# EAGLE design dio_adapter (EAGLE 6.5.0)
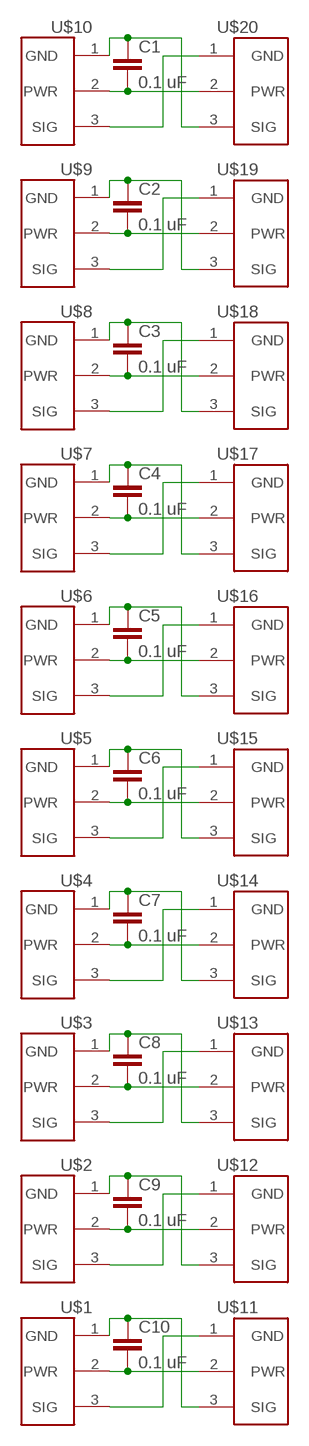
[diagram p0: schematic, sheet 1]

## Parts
C1  0.1 uF  CAP0603  [0603]
C2  0.1 uF  CAP0603  [0603]
C3  0.1 uF  CAP0603  [0603]
C4  0.1 uF  CAP0603  [0603]
C5  0.1 uF  CAP0603  [0603]
C6  0.1 uF  CAP0603  [0603]
C7  0.1 uF  CAP0603  [0603]
C8  0.1 uF  CAP0603  [0603]
C9  0.1 uF  CAP0603  [0603]
C10  0.1 uF  CAP0603  [0603]
U$1  22-23-2031GENERIC  [PWM_1X3]
U$2  22-23-2031GENERIC  [PWM_1X3]
U$3  22-23-2031GENERIC  [PWM_1X3]
U$4  22-23-2031GENERIC  [PWM_1X3]
U$5  22-23-2031GENERIC  [PWM_1X3]
U$6  22-23-2031GENERIC  [PWM_1X3]
U$7  22-23-2031GENERIC  [PWM_1X3]
U$8  22-23-2031GENERIC  [PWM_1X3]
U$9  22-23-2031GENERIC  [PWM_1X3]
U$10  22-23-2031GENERIC  [PWM_1X3]
U$11  22-23-2031  [22-23-2031]
U$12  22-23-2031  [22-23-2031]
U$13  22-23-2031  [22-23-2031]
U$14  22-23-2031  [22-23-2031]
U$15  22-23-2031  [22-23-2031]
U$16  22-23-2031  [22-23-2031]
U$17  22-23-2031  [22-23-2031]
U$18  22-23-2031  [22-23-2031]
U$19  22-23-2031  [22-23-2031]
U$20  22-23-2031  [22-23-2031]

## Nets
N$1: C1.1 U$10.1(GND) U$20.3(SIG)
N$2: C1.2 U$10.2(PWR) U$20.2(PWR)
N$3: U$10.3(SIG) U$20.1(GND)
N$4: C10.1 U$1.1(GND) U$11.3(SIG)
N$5: C2.2 U$9.2(PWR) U$19.2(PWR)
N$6: U$9.3(SIG) U$19.1(GND)
N$7: C9.1 U$2.1(GND) U$12.3(SIG)
N$8: C3.2 U$8.2(PWR) U$18.2(PWR)
N$9: U$8.3(SIG) U$18.1(GND)
N$10: C8.1 U$3.1(GND) U$13.3(SIG)
N$11: C4.2 U$7.2(PWR) U$17.2(PWR)
N$12: U$7.3(SIG) U$17.1(GND)
N$13: C7.1 U$4.1(GND) U$14.3(SIG)
N$14: C5.2 U$6.2(PWR) U$16.2(PWR)
N$15: U$6.3(SIG) U$16.1(GND)
N$16: C6.1 U$5.1(GND) U$15.3(SIG)
N$17: C6.2 U$5.2(PWR) U$15.2(PWR)
N$18: U$5.3(SIG) U$15.1(GND)
N$19: C5.1 U$6.1(GND) U$16.3(SIG)
N$20: C7.2 U$4.2(PWR) U$14.2(PWR)
N$21: U$4.3(SIG) U$14.1(GND)
N$22: C4.1 U$7.1(GND) U$17.3(SIG)
N$23: C8.2 U$3.2(PWR) U$13.2(PWR)
N$24: U$3.3(SIG) U$13.1(GND)
N$25: C3.1 U$8.1(GND) U$18.3(SIG)
N$26: C9.2 U$2.2(PWR) U$12.2(PWR)
N$27: U$2.3(SIG) U$12.1(GND)
N$28: C2.1 U$9.1(GND) U$19.3(SIG)
N$29: C10.2 U$1.2(PWR) U$11.2(PWR)
N$30: U$1.3(SIG) U$11.1(GND)

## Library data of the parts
C1-C10 = custom:CAP: Capacitor
U$1-U$20 = custom:22-23-2031: Molex 3-pin male connector 22-23-2031.

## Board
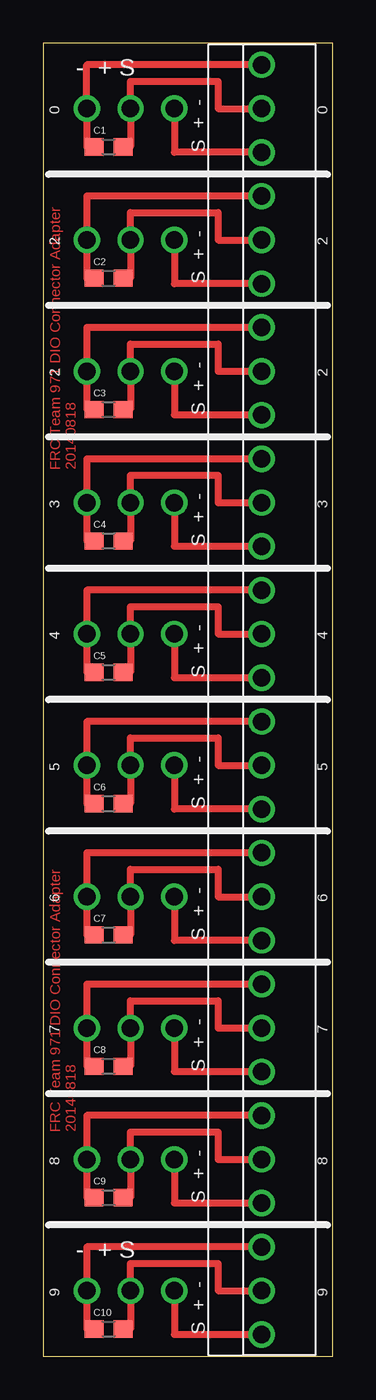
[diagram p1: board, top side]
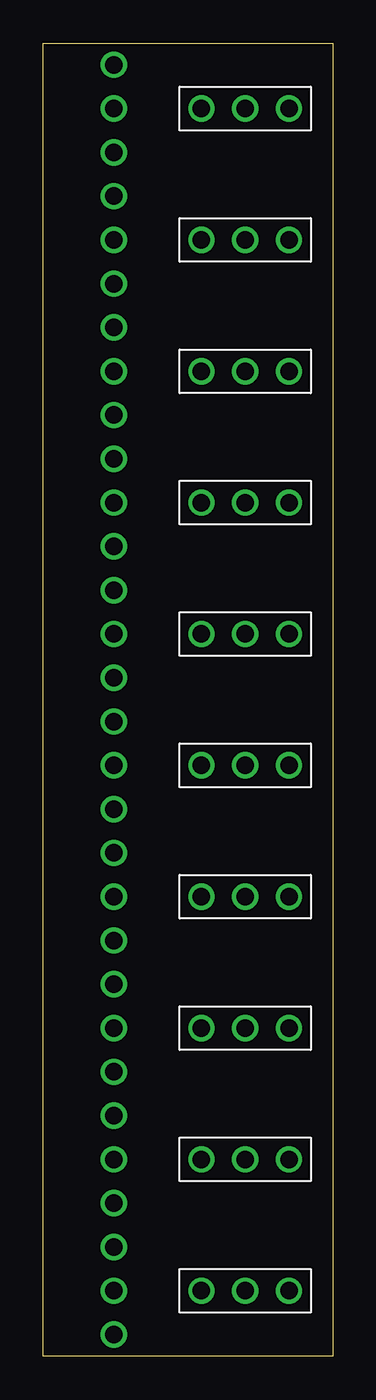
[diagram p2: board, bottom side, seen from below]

Size 16.82 x 76.19 mm. Coordinates in mm from the lower left corner, seen from the top.
Outline: 0,0 16.82,0 16.82,76.19 0,76.19 0,0
Copper layers (1*16): Top 0.035mm / dielectric 1.5mm / Bottom 0.035mm
Design rules "SeeedStudio_2layer_DRU_no_angle_20140221 *": minimum track width 6mil, minimum drill 12mil, track to track 6mil, track to pad 6mil, pad to pad 6mil, via to via 6mil, smd to smd 0mil, copper to edge 10mil, drill to drill 10mil, minimum pad ring 10mil, minimum via ring 6mil, stop-mask expansion 2mil, vias tented up to drill 100mil, thermal gap 10mil

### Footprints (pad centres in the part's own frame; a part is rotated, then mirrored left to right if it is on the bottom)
0603 = smd 1.1 x 1: 1 -0.85,0; 2 0.85,0
PWM_1X3 = drill 1.016: 1 0,2.54; 2 0,0; 3 0,-2.54
22-23-2031 = drill 1.016: 1 0,2.54; 2 0,0; 3 0,-2.54

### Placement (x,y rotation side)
C1  3.81,70.17 0 top
C2  3.81,62.55 0 top
C3  3.81,54.93 0 top
C4  3.81,47.31 0 top
C5  3.81,39.69 0 top
C6  3.81,32.07 0 top
C7  3.81,24.45 0 top
C8  3.81,16.83 0 top
C9  3.81,9.21 0 top
C10  3.81,1.59 0 top
U$1  5.08,3.81 270 bottom
U$2  5.08,11.43 270 bottom
U$3  5.08,19.05 270 bottom
U$4  5.08,26.67 270 bottom
U$5  5.08,34.29 270 bottom
U$6  5.08,41.91 270 bottom
U$7  5.08,49.53 270 bottom
U$8  5.08,57.15 270 bottom
U$9  5.08,64.77 270 bottom
U$10  5.08,72.39 270 bottom
U$11  12.7,3.81 180 top
U$12  12.7,11.43 180 top
U$13  12.7,19.05 180 top
U$14  12.7,26.67 180 top
U$15  12.7,34.29 180 top
U$16  12.7,41.91 180 top
U$17  12.7,49.53 180 top
U$18  12.7,57.15 180 top
U$19  12.7,64.77 180 top
U$20  12.7,72.39 180 top

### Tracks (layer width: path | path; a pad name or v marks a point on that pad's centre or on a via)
N$1
  Top 0.406: C1.1 2.54,70.17 U$10.1 2.54,74.93 U$20.3
N$2
  Top 0.406: U$20.2 10.16,72.39 10.16,73.98 5.08,73.98 U$10.2 5.08,70.17 C1.2
N$3
  Top 0.406: U$10.3 7.62,69.85 U$20.1
N$4
  Top 0.406: C10.1 2.54,1.59 U$1.1 2.54,6.03 2.54,6.35 U$11.3
N$5
  Top 0.406: U$19.2 10.16,64.77 10.16,66.36 5.08,66.36 U$9.2 5.08,62.55 C2.2
N$6
  Top 0.406: U$9.3 7.62,62.23 U$19.1
N$7
  Top 0.406: C9.1 2.54,9.21 U$2.1 2.54,13.97 U$12.3
N$8
  Top 0.406: U$18.2 10.16,57.15 10.16,58.74 5.08,58.74 U$8.2 5.08,54.93 C3.2
N$9
  Top 0.406: U$8.3 7.62,54.61 U$18.1
N$10
  Top 0.406: C8.1 2.54,16.83 U$3.1 2.54,21.59 U$13.3
N$11
  Top 0.406: U$17.2 10.16,49.53 10.16,51.12 5.08,51.12 U$7.2 5.08,47.31 C4.2
N$12
  Top 0.406: U$7.3 7.62,46.99 U$17.1
N$13
  Top 0.406: C7.1 2.54,24.45 U$4.1 2.54,29.21 U$14.3
N$14
  Top 0.406: U$16.2 10.16,41.91 10.16,43.5 5.08,43.5 U$6.2 5.08,39.69 C5.2
N$15
  Top 0.406: U$6.3 7.62,39.37 U$16.1
N$16
  Top 0.406: C6.1 2.54,32.07 U$5.1 2.54,36.83 U$15.3
N$17
  Top 0.406: U$15.2 10.16,34.29 10.16,35.88 5.08,35.88 U$5.2 5.08,32.07 C6.2
N$18
  Top 0.406: U$5.3 7.62,31.75 U$15.1
N$19
  Top 0.406: C5.1 2.54,39.69 U$6.1 2.54,44.45 U$16.3
N$20
  Top 0.406: U$14.2 10.16,26.67 10.16,28.26 5.08,28.26 U$4.2 5.08,24.45 C7.2
N$21
  Top 0.406: U$4.3 7.62,24.13 U$14.1
N$22
  Top 0.406: C4.1 2.54,47.31 U$7.1 2.54,52.07 U$17.3
N$23
  Top 0.406: U$13.2 10.16,19.05 10.16,20.64 5.08,20.64 U$3.2 5.08,16.83 C8.2
N$24
  Top 0.406: U$3.3 7.62,16.51 U$13.1
N$25
  Top 0.406: C3.1 2.54,54.93 U$8.1 2.54,59.69 U$18.3
N$26
  Top 0.406: U$12.2 10.16,11.43 10.16,13.02 5.08,13.02 U$2.2 5.08,9.21 C9.2
N$27
  Top 0.406: U$2.3 7.62,8.89 U$12.1
N$28
  Top 0.406: C2.1 2.54,62.55 U$9.1 2.54,67.31 U$19.3
N$29
  Top 0.406: U$11.2 10.16,3.81 10.16,5.4 5.08,5.4 U$1.2 5.08,1.59 C10.2
N$30
  Top 0.406: U$1.3 7.62,1.27 U$11.1

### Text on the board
Top: FRC Team 971 DIO Connector Adapter / 20140818 | FRC Team 971 DIO Connector Adapter / 20140818
tPlace: - + S | 0 | 0 | S + - | 2 | 2 | S + - | 2 | 2 | S + - | 3 | 3 | S + - | 4 | 4 | S + - | 5 | 5 | S + - | 6 | 6 | S + - | 7 | 7 | S + - | 8 | 8 | S + - | - + S | 9 | 9 | S + -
